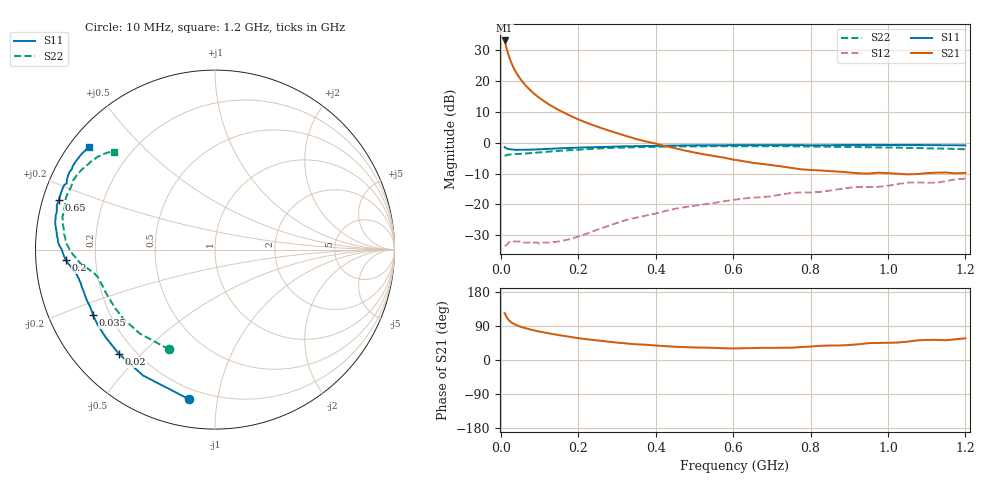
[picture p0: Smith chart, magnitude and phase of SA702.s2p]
!  POLYFET RF DEVICES
!  S PARAMETERS FOR
!  SA702
!  VDS=28, IDQ=400MA
! Date: Tue Aug 29 11:27:30 2000
# MHZ  S  MA  R  50.0000
! SCATTERING PARAMETERS :
! Freq=MHz Mag[s11] Ang[s11] Mag[s21] Ang[s21] Mag[s12] Ang[s12] Mag[s22] Ang[s22]
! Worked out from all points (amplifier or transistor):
!   65 points, 10 MHz to 1.2 GHz, reference 50 ohm
!   highest |S21| = 33.2 dB at 10 MHz (marker M1)
!   |S21| within 3 dB of that: start of sweep to 16.15 MHz
!   unconditionally stable (mu >= 1): 136.3 MHz to 321.6 MHz; 610.2 MHz to end of sweep
!   at 60 MHz: K = 0.47, MSG = 25.8 dB, |S12| = -32.4 dB
!   at 400 MHz: K = 0.98, MSG = 11.3 dB, |S12| = -23.0 dB
!   at 1.2 GHz: K = 1.08, MAG = -0.8 dB, |S12| = -11.7 dB
!   S11 on the Smith chart (normalised r, x): 10 MHz: 0.14, -0.83; 20 MHz: 0.14, -0.43; 35 MHz: 0.14, -0.25; 200 MHz: 0.09, -0.04; 650 MHz: 0.05, +0.15; 1.2 GHz: 0.06, +0.35
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10  0.846 -99.9  45.52 123.8  0.021 36.3  0.612 -114.6
15  0.808 -119.8  34.12 113.1  0.022 28.5  0.628 -132.0
20  0.79 -132.7  26.61 106.2  0.024 23.9  0.639 -142.6
25  0.781 -141.5  21.59 101.2  0.025 22.2  0.645 -149.4
30  0.776 -147.5  18.11 97.5  0.025 21.2  0.648 -154.1
35  0.771 -151.8  15.59 94.7  0.025 19.6  0.652 -157.3
40  0.765 -155.2  13.62 92.4  0.025 19.1  0.656 -159.7
45  0.767 -157.5  12.2 90.2  0.025 17.6  0.657 -161.6
55  0.768 -161.2  9.993 86.6  0.025 19.2  0.664 -164.3
65  0.771 -163.9  8.39 83.7  0.024 19.2  0.67 -166.2
85  0.775 -167.6  6.318 78.4  0.024 22.9  0.683 -168.6
100  0.781 -169.5  5.311 75.0  0.023 28.2  0.696 -170.0
125  0.796 -171.7  4.159 70.2  0.024 37.7  0.718 -171.6
200  0.833 -175.9  2.392 57.8  0.03 62.8  0.77 -175.9
225  0.841 -177.3  2.067 54.4  0.034 69.4  0.787 -177.6
325  0.875 177.3  1.28 43.6  0.056 79.2  0.836 175.8
425  0.894 172.5  0.88 36.5  0.078 81.2  0.864 169.0
625  0.914 163.4  0.504 31.0  0.124 78.3  0.877 157.9
650  0.912 162.4  0.473 31.4  0.128 77.4  0.875 156.5
825  0.905 155.9  0.355 37.4  0.159 75.7  0.863 148.6
1025  0.919 147.9  0.314 46.1  0.214 74.2  0.833 141.5
1200  0.905 140.8  0.324 57.2  0.261 68.2  0.783 135.7
